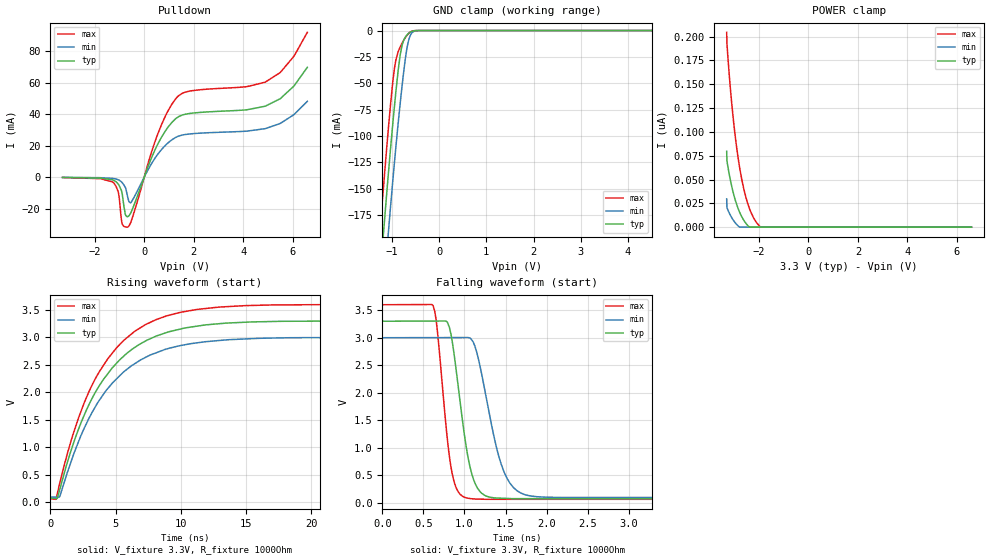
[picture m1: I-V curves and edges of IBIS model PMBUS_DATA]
| Texas Instruments Incorporated
| Digital Controller for Isolated Power
| Part#   Voltage Range   Package_type   #pins
| UCD3138   3.0V - 3.6V   QFN   64
[IBIS ver]   4.0
[File name]   ucd3138.ibs
[File Rev]   2.0
[Date]   10/31/2016
[Source]   Texas Instruments Incorporated.
   Analog_eLab, HPA
   12500 TI Blvd
   Dallas, TX _75243
[Notes]   Revision History
   Rev 1.0: 10/31/2016
   - PMBUS_DATA mdoel(I/O open drain) added, replacing the old
   incorrect push-pull model.
   Rev 1.0: 11/18/2015
   - Initial version of the model
   - Model based on simulations from Spectre
   - Model not matched to measurements
   - Non_monotonic behavior is as per buffer simulations
[Disclaimer] This model is designed as an aid for customers of Texas Instruments.
 TI and its licensors and suppliers make no warranties, either expressed
 or implied, with respect to this  model, including the warranties of
 merchantability or fitness for a particular purpose.
 The model is provided solely on an "as is" basis. The entire risk as to
 its quality and performance is with the customer.
[Copyright] (C)Copyright 2010 Texas Instruments Incorporated.
   All rights reserved.
|   Component UCD3138
[Component]   UCD3138
[Manufacturer]  Texas Instruments Incorporated
[Package]  |QFN   64
|   typ   min   max
R_pkg   0.067   0.027   0.083
L_pkg   0.937nH   0.593nH   1.143nH
C_pkg   0.144pF   0.126pF   0.200pF
[Pin] signal_name   model_name   R_pin   L_pin   C_pin
1   AGND   GND   NA   NA   NA
2   AD13   TERM   NA   NA   NA
3   AD12   TERM   NA   NA   NA
4   AD10   TERM   NA   NA   NA
5   AD07   TERM   NA   NA   NA
6   AD06   TERM   NA   NA   NA
7   AD04   TERM   NA   NA   NA
8   AD03   TERM   NA   NA   NA
9   V33DIO   POWER   NA   NA   NA
10   DGND   GND   NA   NA   NA
11   RESTB   TERM   NA   NA   NA
12   ADC_EXT_TRIG   TERM   NA   NA   NA
13   SCI_RX0   TERM   NA   NA   NA
14   SCI_TX0   TERM   NA   NA   NA
15   PMBUS_CLK   PMBUS_DATA   NA   NA   NA
16   PMBUS_DATA   PMBUS_DATA   NA   NA   NA
17   DPWM0A   TERM   NA   NA   NA
18   DPWM0B   TERM   NA   NA   NA
19   DPWM1A   TERM   NA   NA   NA
20   DPWM1B   TERM   NA   NA   NA
21   DPWM2A   TERM   NA   NA   NA
22   DPWM2B   TERM   NA   NA   NA
23   DPWM3A   TERM   NA   NA   NA
24   DPWM3B   TERM   NA   NA   NA
25   DGND   GND   NA   NA   NA
26   SNC   TERM   NA   NA   NA
27   PMBUS_ALERT   TERM   NA   NA   NA
28   PMBUS_CTRL   TERM   NA   NA   NA
29   SCI_TX1   TERM   NA   NA   NA
30   SCI_RX1   TERM   NA   NA   NA
31   PWM0   TERM   NA   NA   NA
32   PWM1   TERM   NA   NA   NA
33   DGND   GND   NA   NA   NA
34   IN_EXT   TERM   NA   NA   NA
35   FAULT0   TERM   NA   NA   NA
36   FAULT1   TERM   NA   NA   NA
37   TCK   TERM   NA   NA   NA
38   TDO   TERM   NA   NA   NA
39   TDI   TERM   NA   NA   NA
40   TMS   TERM   NA   NA   NA
41   TCAP   TERM   NA   NA   NA
42   FAULT2   TERM   NA   NA   NA
43   FAULT3   TERM   NA   NA   NA
44   DGND   GND   NA   NA   NA
45   V33DIO   POWER   NA   NA   NA
46   BP18   TERM   NA   NA   NA
47   V33D   POWER   NA   NA   NA
48   AGND   GND   NA   NA   NA
49   AGND   GND   NA   NA   NA
50   EAP0   TERM   NA   NA   NA
51   EAN0   TERM   NA   NA   NA
52   EAP1   TERM   NA   NA   NA
53   EAN1   TERM   NA   NA   NA
54   EAP2   TERM   NA   NA   NA
55   EAN2   TERM   NA   NA   NA
56   AGND   GND   NA   NA   NA
57   V33A   POWER   NA   NA   NA
58   AD00   TERM   NA   NA   NA
59   AD01   TERM   NA   NA   NA
60   AD02   TERM   NA   NA   NA
61   AD05   TERM   NA   NA   NA
62   AD08   TERM   NA   NA   NA
63   AD09   TERM   NA   NA   NA
64   AD11   TERM   NA   NA   NA
[Model] TERM
Model_type Terminator
C_comp   0  0  0
| variable   typ   min   max
[Voltage Range]   3.30000V  3.00000V  3.60000V
[POWER Clamp Reference]  3.30000V  3.00000V  3.60000V
[GND Clamp Reference]   0.00000V  0.00000V  0.00000V
[Temperature Range]   27   110   -40
| Models and submodels in the file (2): TERM (Terminator), PMBUS_DATA (I/O_open_drain)
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|   PMBUS_DATA 3.3V Model
[Model]   PMBUS_DATA
Model_type   I/O_open_drain
Polarity   Non-Inverting
Enable   Active-Low
Vinl = 1.1
Vinh = 2.1
Vmeas = 1.65
Vref = 3.3
Cref = 1pF
Rref = 1000
|   typ   min   max
C_comp   1pF   1pF   1pF
[Voltage Range]   3.3   3   3.6
[Temperature Range]   27   110   -40
[Pullup Reference]   3.3   3   3.6
[Pulldown Reference]   -0   -0   -0
[Power Clamp Reference]   3.3   3   3.6
[GND Clamp Reference]   -0   -0   -0
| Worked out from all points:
|   slope of the pulldown table from 0 to 0.495 V, typ, clamps not added: 25.6 ohm
|   GND clamp passes 1 mA (typ) near -0.59 V on its own axis
|   falling waveform, V_fixture 3.3V, R_fixture 1000Ohm: 20-80 % time 180ps typ, 255ps min, 138ps max; typ from 3.3 V to 0.072 V
|   rising waveform, V_fixture 3.3V, R_fixture 1000Ohm: 20-80 % time 4.3ns typ, 4.36ns min, 4.22ns max; typ from 0.072 V to 3.3 V
[Pulldown]
|   Voltage   I(typ)   I(min)   I(max)
-3.3V     -161.6uA   -95.67uA   -239.5uA
-1.28V    -1.688mA   -780.9uA   -3.006mA
-1.043V   -4.549mA   -1.684mA   -9.829mA
-884.4mV  -11.01mA   -3.591mA   -29.97mA
-765.6mV  -23.48mA   -6.398mA   -31.6mA
-656.7mV  -25.05mA   -13.37mA   -31.63mA
-518.1mV  -21.9mA    -15.78mA   -27.67mA
561mV     21.41mA    14.86mA    28.02mA
1.323V    37.81mA    25.68mA    50.76mA
4.887V    45.12mA    30.85mA    60.42mA
5.511V    50.12mA    34.31mA    66.83mA
6.59V     69.87mA    48.23mA    92.11mA
[GND Clamp]
|   Voltage   I(typ)   I(min)   I(max)
-3.3V     -1.479A    -1.52A     -1.447A
-1.261V   -239.9mA   -295.8mA   -196mA
-1.191V   -200.6mA   -256.8mA   -156.7mA
-1.073V   -135.8mA   -191.5mA   -92.9mA
-983.4mV  -90.47mA   -144.9mA   -50.45mA
-943.8mV  -71.69mA   -125.1mA   -35.8mA
-825mV    -24.03mA   -70.22mA   -15.79mA
-765.6mV  -11.57mA   -45.93mA   -10.55mA
-696.3mV  -5.224mA   -21.46mA   -5.541mA
-646.8mV  -2.766mA   -9.894mA   -2.862mA
-587.4mV  -983.3uA   -3.003mA   -890.3uA
6.59V     0A         0A         0A
[POWER Clamp]
|   Voltage   I(typ)   I(min)   I(max)
-3.3V     79.58nA    29.7nA     204.5nA
-3.29V    69.72nA    20.6nA     192.8nA
-3.251V   63.41nA    18.06nA    178.4nA
-3.161V   50.81nA    13.07nA    149nA
-3.072V   40.14nA    8.944nA    123.6nA
-2.924V   26nA       3.641nA    88.97nA
-2.756V   14.39nA    0A         59.34nA
-2.587V   6.336nA    0A         37.76nA
-2.369V   0A         0A         18.8nA
-2.211V   0A         0A         9.654nA
-1.944V   0A         0A         189.8pA
6.59V     0A         0A         0A
[Ramp]
R_load = 1000
|   typ   min   max
dV/dt_r   1.93678/4.28869e-09   1.74422/4.35666e-09   2.12337/4.22655e-09
dV/dt_f   1.93678/1.79918e-10   1.74422/2.54903e-10   2.12337/1.37977e-10
[Falling Waveform]
V_fixture = 3.3V
V_fixture_min = 3V
V_fixture_max = 3.6V
R_fixture = 1000Ohm
C_fixture = 0F
|   Time   V(typ)   V(min)   V(max)
0s        3.3V       3V         3.6V
617.7ps   3.303V     3.002V     3.582V
667.7ps   3.304V     3.002V     3.152V
791.7ps   3.281V     3.003V     1.153V
894.3ps   2.463V     3.003V     288.1mV
1.064ns   669.3mV    2.995V     75.29mV
1.259ns   123.6mV    1.953V     61.81mV
1.553ns   75.2mV     355.7mV    61.81mV
2.172ns   73.59mV    94.98mV    61.81mV
200ns     72.03mV    92.96mV    61.06mV
[Rising Waveform]
V_fixture = 3.3V
V_fixture_min = 3V
V_fixture_max = 3.6V
R_fixture = 1000Ohm
C_fixture = 0F
|   Time   V(typ)   V(min)   V(max)
0s        72.03mV    92.96mV    61.06mV
429.4ps   64.2mV     90.24mV    51.25mV
728.9ps   232.4mV    102.5mV    348mV
1.72ns    1.033V     825.7mV    1.218V
2.956ns   1.773V     1.524V     2.01V
4.042ns   2.227V     1.955V     2.481V
5.071ns   2.53V      2.245V     2.811V
8.102ns   3.025V     2.721V     3.326V
12.92ns   3.251V     2.945V     3.554V
200ns     3.3V       3V         3.6V
